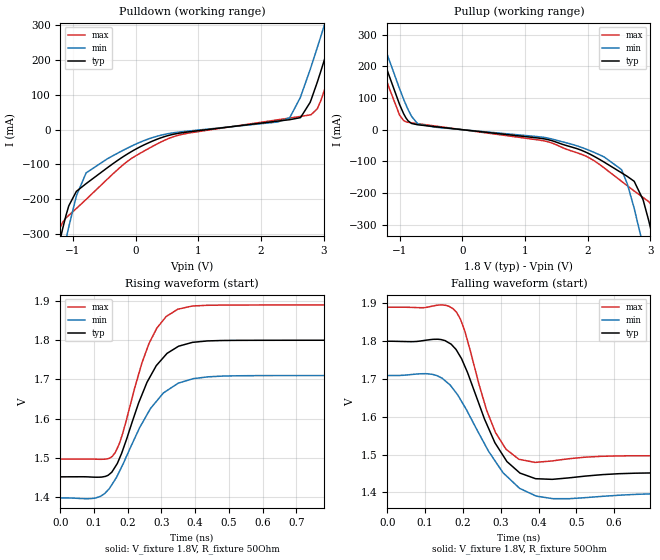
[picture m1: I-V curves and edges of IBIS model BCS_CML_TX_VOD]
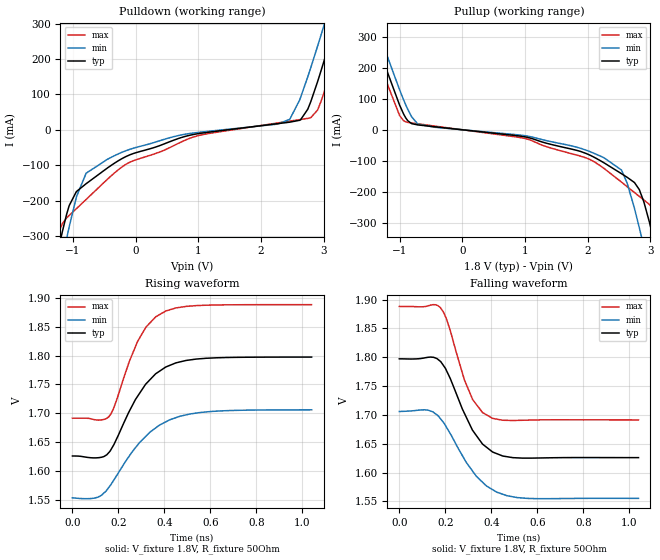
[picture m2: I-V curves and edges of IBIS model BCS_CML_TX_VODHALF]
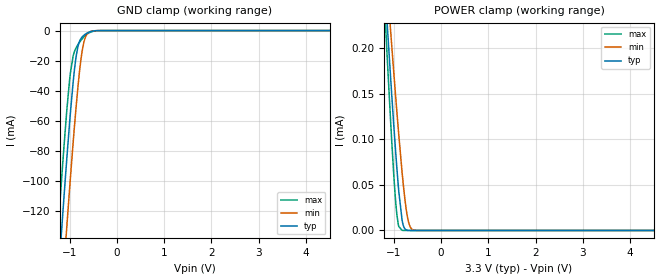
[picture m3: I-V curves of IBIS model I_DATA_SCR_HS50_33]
| Texas Instruments Incorporated
| DS90UB903Q
| 10-43-MHz 18-Bit Color FPD Link III Serializer and Deserializer
| with Bi-Directional Control Channel
| Marketing part#   Voltage Range   Package-type   Temperature
| DS92LX2121SQE   1.71V - 3.6V   40-Pin LLP   -40 to 105C
| DS92LX2121SQ   1.71V - 3.6V   40-Pin LLP   -40 to 105C
| DS92LX2121SQX   1.71V - 3.6V   40-Pin LLP   -40 to 105C
[IBIS Ver]   4.0
[File name]   ds92lx2121.ibs
[File Rev]   1.0
[Date]   04/11/2012
[Source]   Model built from TISPICE simulations at:
   Texas Instruments Incorporated.
   WEBENCH DESIGN CENTER
   12500 TI Blvd
   Dallas, TX -75243
   For Support e-mail: elab_scm_ibis@list.ti.com
[Notes]   Rev 1.0: 04/11/2012
   - Initial version of the IBIS model
   - All models are generated in Spectre
   - ccomp is listed in numerical order, for PVT information,
   please check notes above ccomp keyword for each model
   - All non-monotonic warnings can be ignored as per buffer behavior
[Disclaimer] This product is designed as an aid for customers of Texas Instruments.
   No warranties, either expressed or implied, with respect to this third
   party software (if any) or with respect to its fitness for any
   particular purpose is claimed by Texas Instruments or the author. The
   software (if any) is provided solely on an "as is" basis. The entire
   risk as to its quality and performance is with the customer
[Copyright]   (C)Copyright 2012 Texas Instruments Incorporated.
   All rights reserved.
|   DS92LX2121
[Component]  DS92LX2121
[Manufacturer]  Texas Instruments, Inc.
[Package]   |40-pin LLP 7.0x7.0x0.5mm
|   typ   min   max
R_pkg   0   0   0
L_pkg   0   0   0
C_pkg   0   0   0
[Pin]   signal_name   model_name   R_pin   L_pin   C_pin
1   DIN[16]   I_DATA_SCR_HS50
2   DIN[17]   I_DATA_SCR_HS50
3   DIN[18]   I_DATA_SCR_HS50
4   DIN[19]   I_DATA_SCR_HS50
5   DIN[20]   I_DATA_SCR_HS50
6   PCLK   IO_CLK_50_HS50
7   SCL   IO_SMBUS_HS50
8   SDA   IO_SMBUS_HS50
9   ID[x]   NC
10   RES   NC
11   RES   NC
12   MODE   I_PWDN_SCR_HS50
13   PDB   I_PWDN_SCR_HS50
14   VDDPLL   POWER
15   VDDT   POWER
16   DOUT-   BCS_CML_TX
17   DOUT+   BCS_CML_TX
18   VDDCML   POWER
19   GPO[0]   IO_DATA_50_ATP_HS50
20   GPO[1]   IO_DATA_50_ATP_HS50
21   GPO[2]   IO_DATA_50_ATP_HS50
22   GPO[3]   IO_DATA_50_ATP_HS50
23   DIN[0]   IO_DATA_50_HS50
24   DIN[1]   IO_DATA_50_HS50
25   DIN[2]   IO_DATA_50_ATP_HS50
26   DIN[3]   IO_DATA_50_ATP_HS50
27   DIN[4]   I_DATA_SCR_HS50
28   DIN[5]   I_DATA_SCR_HS50
29   DIN[6]   I_DATA_SCR_HS50
30   DIN[7]   I_DATA_SCR_HS50
31   VDDIO   POWER
32   DIN[8]   I_DATA_SCR_HS50
33   DIN[9]   I_DATA_SCR_HS50
34   VDDD   POWER
35   DIN[10]   I_DATA_SCR_HS50
36   DIN[11]   I_DATA_SCR_HS50
37   DIN[12]   I_DATA_SCR_HS50
38   DIN[13]   I_DATA_SCR_HS50
39   DIN[14]   I_DATA_SCR_HS50
40   DIN[15]   I_DATA_SCR_HS50
41   DAP   GND
[Package Model] llp40_DS92LX2121
[Diff Pin]  inv_pin  vdiff  tdelay_typ tdelay_min tdelay_max
17   16   NA   NA   NA   NA
[Model Selector]   I_DATA_SCR_HS50
I_DATA_SCR_HS50_33   I_DATA_SCR_HS50 input with VDD=3.3V
I_DATA_SCR_HS50_18   I_DATA_SCR_HS50 input with VDD=1.8V
[Model Selector]   I_PWDN_SCR_HS50
I_PWDN_SCR_HS50_33   I_PWDN_SCR_HS50 input with VDD=3.3V
I_PWDN_SCR_HS50_18   I_PWDN_SCR_HS50 input with VDD=1.8V
[Model Selector]   IO_DATA_50_ATP_HS50
IO_DATA_50_ATP_HS50_33   IO_DATA_50_ATP_HS50 with VDD=3.3V
IO_DATA_50_ATP_HS50_18   IO_DATA_50_ATP_HS50 with VDD=1.8V
[Model Selector]   IO_DATA_50_HS50
IO_DATA_50_HS50_33   IO_DATA_50_HS50 with VDD=3.3V
IO_DATA_50_HS50_18   IO_DATA_50_HS50 with VDD=1.8V
[Model Selector]   IO_SMBUS_HS50
IO_SMBUS_HS50_33   IO_SMBUS_HS50 with VDD=3.3V
IO_SMBUS_HS50_18   IO_SMBUS_HS50 with VDD=1.8V
[Model Selector]   IO_CLK_50_HS50
IO_CLK_50_HS50_33   IO_CLK_50_HS50 with VDD=3.3V
IO_CLK_50_HS50_18   IO_CLK_50_HS50 with VDD=1.8V
[Model Selector]   BCS_CML_TX
BCS_CML_TX_VOD   CML driver with full swing
BCS_CML_TX_VODHALF   CML driver with hafl swing
|   Package model for DS90UB903
[Define Package Model]  llp40_DS92LX2121
[Manufacturer]  Texas Instruments,Inc.
[OEM]  Texas Instruments,Inc.
[Description]  Package model with Au wires, simulation frequency of 1.4GHz,
|Buildsheet#DS90UB903QSQ-04 RevA
[Number Of Pins]  41
[Pin Numbers]
41   | 41 = DAP
1   | 1 = L1
2   | 2 = L2
3   | 3 = L3
4   | 4 = L4
5   | 5 = L5
6   | 6 = L6
7   | 7 = L7
8   | 8 = L8
9   | 9 = L9
10   | 10 = L10
11   | 11 = L11
12   | 12 = L12
13   | 13 = L13
14   | 14 = L14
15   | 15 = L15
16   | 16 = L16
17   | 17 = L17
18   | 18 = L18
19   | 19 = L19
20   | 20 = L20
21   | 21 = L21
22   | 22 = L22
23   | 23 = L23
24   | 24 = L24
25   | 25 = L25
26   | 26 = L26
27   | 27 = L27
28   | 28 = L28
29   | 29 = L29
30   | 30 = L30
31   | 31 = L31
32   | 32 = L32
33   | 33 = L33
34   | 34 = L34
35   | 35 = L35
36   | 36 = L36
37   | 37 = L37
38   | 38 = L38
39   | 39 = L39
40   | 40 = L40
[Model Data]
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[End Model Data]
[End Package Model]
| Models and submodels in the file (14): BCS_CML_TX_VOD (Output), BCS_CML_TX_VODHALF (Output), I_DATA_SCR_HS50_33 (Input), I_DATA_SCR_HS50_18 (Input), I_PWDN_SCR_HS50_33 (Input), I_PWDN_SCR_HS50_18 (Input), IO_DATA_50_ATP_HS50_33 (I/O), IO_DATA_50_ATP_HS50_18 (I/O), IO_DATA_50_HS50_33 (I/O), IO_DATA_50_HS50_18 (I/O), IO_SMBUS_HS50_33 (I/O_open_drain), IO_SMBUS_HS50_18 (I/O_open_drain), IO_CLK_50_HS50_33 (I/O), IO_CLK_50_HS50_18 (I/O)
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|   Model BCS_CML_TX_VOD
[Model]   BCS_CML_TX_VOD
Model_type   Output
Polarity   Non-Inverting
Vmeas = 1.65
Vref = 1.8
Cref = 1pF
Rref = 50
|   typ   min   max
C_comp   1.327pF   1.280pF   1.352pF
[Voltage Range]   1.8   1.71   1.89
[Temperature Range]   25   105   -40
[Pullup Reference]   1.8   1.71   1.89
[Pulldown Reference]   0   0   0
[Power Clamp Reference]   1.8   1.71   1.89
[GND Clamp Reference]   0   0   0
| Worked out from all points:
|   slope of the pulldown table from 0 to 0.27 V, typ, clamps not added: 11.6 ohm
|   slope of the pullup table from 0 to 0.27 V, typ, clamps not added: 46.1 ohm
|   falling waveform, V_fixture 1.8V, R_fixture 50Ohm: 20-80 % time 84.6ps typ, 108ps min, 70.1ps max; typ from 1.8 V to 1.45 V
|   rising waveform, V_fixture 1.8V, R_fixture 50Ohm: 20-80 % time 95.8ps typ, 116ps min, 85.6ps max; typ from 1.45 V to 1.8 V
[Pulldown]
|   Voltage   I(typ)   I(min)   I(max)
-1.8V     -861.7mA   -948.5mA   -797.6mA
-1.201V   -312.8mA   -391.7mA   -279.8mA
-1.114V   -248.1mA   -317.9mA   -254.3mA
-790.2mV  -155mA     -124.1mA   -200.4mA
68.4mV    -49.54mA   -36.17mA   -68.12mA
716.4mV   -9.411mA   -6.34mA    -14.36mA
2.461V    28.87mA    34.58mA    33.61mA
2.633V    35.08mA    94.78mA    38.23mA
2.801V    85.68mA    181mA      43.26mA
2.957V    168.8mA    268.9mA    84.2mA
3.103V    253.7mA    353.2mA    164mA
3.595V    553.3mA    645.1mA    468.7mA
[Pullup]
|   Voltage   I(typ)   I(min)   I(max)
-1.8V     551mA      589.5mA    522.5mA
-1.238V   209.3mA    258.5mA    171.2mA
-936mV    49.07mA    94.45mA    28.3mA
-714.6mV  15.55mA    18.58mA    19.05mA
1.294V    -28.58mA   -24.09mA   -34.98mA
1.894V    -64.55mA   -55.41mA   -77.27mA
2.536V    -135.7mA   -125.6mA   -162.4mA
2.741V    -163.1mA   -248.7mA   -193.5mA
2.882V    -220.7mA   -365mA     -213.7mA
3.049V    -350.2mA   -514.5mA   -245.7mA
3.233V    -514.3mA   -684.8mA   -372.3mA
3.595V    -855.8mA   -1.029A    -705.1mA
[Ramp]
R_load = 50
|   typ   min   max
dV/dt_r   0.209023/9.57522e-11   0.187159/1.16048e-10   0.235879/8.5583e-11
dV/dt_f   0.209162/8.46157e-11   0.186888/1.07876e-10   0.236093/7.00733e-11
[Falling Waveform]
V_fixture = 1.8V
V_fixture_min = 1.71V
V_fixture_max = 1.89V
R_fixture = 50Ohm
C_fixture = 0F
|   Time   V(typ)   V(min)   V(max)
0s        1.8V       1.709V     1.89V
118.8ps   1.805V     1.712V     1.893V
183.5ps   1.775V     1.661V     1.876V
205.1ps   1.734V     1.626V     1.827V
262.5ps   1.582V     1.518V     1.618V
285.9ps   1.529V     1.482V     1.559V
313.8ps   1.486V     1.445V     1.514V
348ps     1.453V     1.412V     1.487V
438ps     1.435V     1.383V     1.483V
1.04ns    1.451V     1.398V     1.497V
[Rising Waveform]
V_fixture = 1.8V
V_fixture_min = 1.71V
V_fixture_max = 1.89V
R_fixture = 50Ohm
C_fixture = 0F
|   Time   V(typ)   V(min)   V(max)
0s        1.452V     1.398V     1.497V
103.5ps   1.451V     1.397V     1.497V
154ps     1.466V     1.434V     1.504V
183.5ps   1.516V     1.48V      1.559V
241.8ps   1.661V     1.587V     1.742V
262.5ps   1.701V     1.619V     1.791V
313.8ps   1.764V     1.67V      1.86V
348ps     1.783V     1.69V      1.879V
482ps     1.799V     1.709V     1.89V
1.04ns    1.8V       1.71V      1.89V
|   Model BCS_CML_TX_VOD_HALF
[Model]   BCS_CML_TX_VODHALF
Model_type   Output
Polarity   Non-Inverting
Vmeas = 1.7
Vref = 1.8
Cref = 1pF
Rref = 50
|   typ   min   max
C_comp   1.327pF   1.280pF   1.352pF
[Voltage Range]   1.8   1.71   1.89
[Temperature Range]   25   105   -40
[Pullup Reference]   1.8   1.71   1.89
[Pulldown Reference]   0   0   0
[Power Clamp Reference]   1.8   1.71   1.89
[GND Clamp Reference]   0   0   0
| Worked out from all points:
|   slope of the pulldown table from 0 to 0.27 V, typ, clamps not added: 20.1 ohm
|   slope of the pullup table from 0 to 0.27 V, typ, clamps not added: 45.7 ohm
|   falling waveform, V_fixture 1.8V, R_fixture 50Ohm: 20-80 % time 121ps typ, 147ps min, 95.1ps max; typ from 1.8 V to 1.63 V
|   rising waveform, V_fixture 1.8V, R_fixture 50Ohm: 20-80 % time 151ps typ, 186ps min, 120ps max; typ from 1.63 V to 1.8 V
[Pulldown]
|   Voltage   I(typ)   I(min)   I(max)
-1.8V     -861.6mA   -948.3mA   -797.5mA
-1.195V   -307.7mA   -386.7mA   -275.1mA
-1.103V   -239.7mA   -308.5mA   -248.9mA
-790.2mV  -152.1mA   -122.5mA   -196.5mA
-223.2mV  -81.75mA   -63.72mA   -105.5mA
986.4mV   -11.14mA   -7.555mA   -16.98mA
2.461V    21.67mA    29.69mA    24.58mA
2.633V    28.5mA     91.58mA    29.2mA
2.795V    79.24mA    175.3mA    34.18mA
3.011V    196.7mA    297.3mA    107.6mA
3.114V    257.1mA    357mA      166.5mA
3.595V    550.5mA    642.7mA    465.3mA
[Pullup]
|   Voltage   I(typ)   I(min)   I(max)
-1.8V     551.2mA    589.7mA    522.8mA
-1.238V   209.5mA    258.7mA    171.5mA
-936mV    49.33mA    94.63mA    28.8mA
-714.6mV  15.9mA     18.84mA    19.48mA
986.4mV   -22.21mA   -18.54mA   -27.33mA
1.98V     -76.74mA   -66.02mA   -90.91mA
2.536V    -141mA     -129.3mA   -168.1mA
2.822V    -192.5mA   -315.3mA   -214.4mA
2.893V    -230.6mA   -375.2mA   -225.5mA
3.055V    -356mA     -520mA     -257.3mA
3.244V    -524.9mA   -695.3mA   -384mA
3.595V    -856.1mA   -1.029A    -705.9mA
[Ramp]
R_load = 50
|   typ   min   max
dV/dt_r   0.102748/1.51441e-10  0.0913928/1.85584e-10   0.117926/1.20421e-10
dV/dt_f   0.102771/1.20609e-10  0.0903412/1.47113e-10   0.117973/9.51354e-11
[Falling Waveform]
V_fixture = 1.8V
V_fixture_min = 1.71V
V_fixture_max = 1.89V
R_fixture = 50Ohm
C_fixture = 0F
|   Time   V(typ)   V(min)   V(max)
0s        1.797V     1.706V     1.888V
125.7ps   1.8V       1.708V     1.889V
178.2ps   1.793V     1.694V     1.886V
205.1ps   1.777V     1.679V     1.867V
283ps     1.703V     1.624V     1.761V
319.3ps   1.673V     1.602V     1.726V
362ps     1.649V     1.583V     1.704V
406ps     1.636V     1.57V      1.694V
555.5ps   1.625V     1.555V     1.691V
1.04ns    1.626V     1.555V     1.691V
[Rising Waveform]
V_fixture = 1.8V
V_fixture_min = 1.71V
V_fixture_max = 1.89V
R_fixture = 50Ohm
C_fixture = 0F
|   Time   V(typ)   V(min)   V(max)
0s        1.626V     1.554V     1.692V
111ps     1.623V     1.555V     1.688V
157.3ps   1.632V     1.571V     1.694V
178.2ps   1.644V     1.583V     1.708V
247ps     1.703V     1.626V     1.789V
283ps     1.729V     1.645V     1.824V
319.3ps   1.751V     1.66V      1.849V
406ps     1.78V      1.685V     1.877V
599.5ps   1.796V     1.703V     1.887V
1.04ns    1.797V     1.706V     1.888V
|   Model I_DATA_SCR_HS50_33
[Model] I_DATA_SCR_HS50_33
Model_type Input
Vinl =   0.8
Vinh =   2.0
|   typ   min   max
|   (nom)   (slow)   (fast)
C_comp   0.3665pF   0.3665pF   0.3665pF
[Temperature Range]   25.000   105.000   -40.000
[Voltage Range]   3.300V   3.0000V   3.6000V
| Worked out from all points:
|   GND clamp passes 1 mA (typ) near -0.58 V on its own axis
|   POWER clamp passes 1 mA (typ) near -2.02 V on its own axis
[GND Clamp]
|   Voltage   I(typ)   I(min)   I(max)
-3.3V     -1.166A    -1.209A    -1.134A
-1.32V    -202.1mA   -249mA     -167.1mA
-1.241V   -165.6mA   -212.4mA   -130.7mA
-1.142V   -121mA     -167.4mA   -86.89mA
-1.063V   -86.78mA   -132.3mA   -54.56mA
-983.4mV  -54.93mA   -98.36mA   -28.27mA
-924mV    -33.98mA   -74.16mA   -16.74mA
-825mV    -10.8mA    -38mA      -9.446mA
-755.7mV  -5.134mA   -18.34mA   -6.356mA
-696.3mV  -3.098mA   -7.601mA   -4.22mA
-567.6mV  -815.5uA   -746uA     -1.217mA
6.59V     0A         0A         0A
[POWER Clamp]
|   Voltage   I(typ)   I(min)   I(max)
-3.3V     2.159mA    1.892mA    2.559mA
-1.191V   270.3uA    306.6uA    243.1uA
-1.132V   220.6uA    264.4uA    182.9uA
-1.063V   164.1uA    216.1uA    115.7uA
-993.3mV  110.2uA    168.9uA    55.28uA
-933.9mV  67.72uA    129.8uA    16.89uA
-894.3mV  42.8uA     104.8uA    4.336uA
-825mV    11.61uA    64.2uA     166.8nA
-755.7mV  1.271uA    30.48uA    2.122nA
-696.3mV  130.3nA    11.15uA    0A
-557.7mV  0A         260.4nA    0A
6.59V     0A         0A         0A
